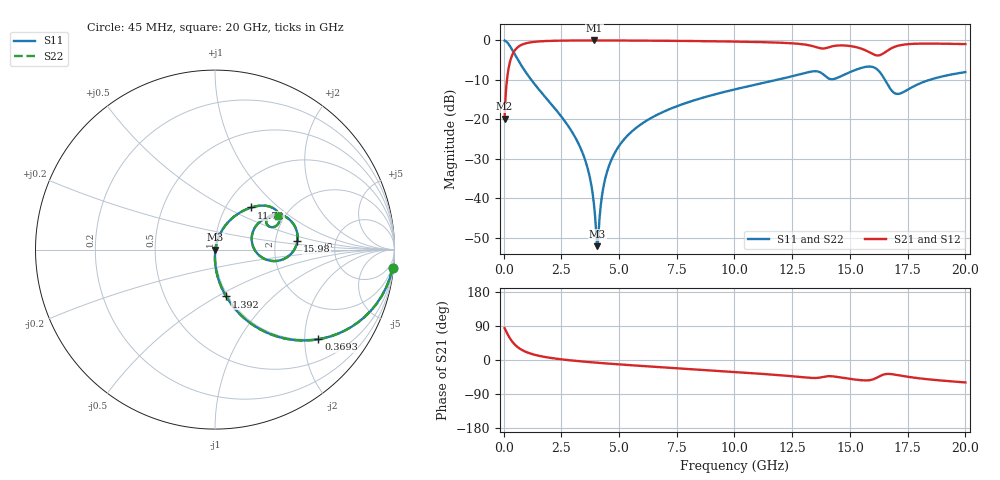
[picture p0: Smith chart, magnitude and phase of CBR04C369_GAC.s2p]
! S-parameter model data by Modelithics Inc.  support@modelithics.com 813-866-6335  Tampa FL USA
! S-Parameter data specifications:
! Substrate: 20-mil Rogers 4350B, substrate thickness, H=0.508mm, Dielectric constant, Er=3.75
! PCB Mounting Pad Footprint: Pad width, PadW=0.52mm , Pad length, PadL=0.52mm , Pad gap, PadG (edge-to-edge)=0.28mm , Reference planes=1.32mm apart
#  GHz  S  MA  R 50
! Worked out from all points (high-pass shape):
!   801 points, 45 MHz to 20 GHz, reference 50 ohm
!   highest |S21| = -0.02 dB at 3.936 GHz (marker M1); lowest = -19.8 dB at 45 MHz (marker M2)
!   |S21| within 3 dB of the highest: 433.5 MHz to 15.84 GHz (15.41 GHz wide, 189 % of centre); 16.52 GHz to end of sweep
!   lowest |S11| = -52.1 dB at 4.061 GHz (marker M3), VSWR 1.00, Z = 50.2 - j0.0389 ohm
!   |S11| at or under -10 dB: 1.202 GHz to 11.83 GHz (10.63 GHz wide, 163 % of centre); 16.52 GHz to 18.45 GHz (1.929 GHz wide, 11 % of centre)
!   |S22| runs from -52.1 to 0.0 dB; largest |S21 - S12| = 0
!   S11 on the Smith chart (normalised r, x): 45 MHz: 1, -19; 369.3 MHz: 0.97, -2.33; 1.392 GHz: 0.98, -0.55; 11.72 GHz: 1.31, +0.68; 15.98 GHz: 2.67, +0.32; 20 GHz: 1.85, +0.81
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0.045  0.9948 -5.9  0.102 84.1  0.102 84.1  0.9948 -5.9
0.219606  0.8937 -27.0  0.4484 62.9  0.4484 62.9  0.8937 -27.0
0.369269  0.7624 -40.9  0.6466 49.0  0.6466 49.0  0.7624 -40.9
0.768369  0.4822 -62.4  0.875 27.5  0.875 27.5  0.4822 -62.4
1.391962  0.2682 -76.6  0.9619 13.1  0.9619 13.1  0.2682 -76.6
3.387462  0.03982 -90.5  0.9968 -3.8  0.9968 -3.8  0.03982 -90.5
3.736675  0.01841 -88.2  0.9973 -5.6  0.9973 -5.6  0.01841 -88.2
3.936225  0.007312 -77.1  0.9974 -6.6  0.9974 -6.6  0.007312 -77.1
4.060944  0.002488 -8.9  0.9974 -7.3  0.9974 -7.3  0.002488 -8.9
4.385212  0.01698 72.4  0.9971 -8.8  0.9971 -8.8  0.01698 72.4
4.784313  0.03621 75.1  0.9965 -10.6  0.9965 -10.6  0.03621 75.1
5.532625  0.06939 73.7  0.9945 -13.9  0.9945 -13.9  0.06939 73.7
6.704981  0.1165 69.7  0.9897 -18.7  0.9897 -18.7  0.1165 69.7
10.0225  0.24 56.9  0.9651 -31.8  0.9651 -31.8  0.24 56.9
11.71867  0.3107 49.1  0.94 -39.0  0.94 -39.0  0.3107 49.1
13.36496  0.4042 33.0  0.8488 -47.3  0.8488 -47.3  0.4042 33.0
14.26294  0.3226 27.3  0.8444 -43.2  0.8444 -43.2  0.3226 27.3
15.23574  0.4224 26.7  0.8248 -51.7  0.8248 -51.7  0.4224 26.7
15.98406  0.4611 5.9  0.6717 -51.4  0.6717 -51.4  0.4611 5.9
16.68248  0.261 -9.1  0.7609 -36.8  0.7609 -36.8  0.261 -9.1
17.13147  0.211 13.9  0.8618 -40.5  0.8618 -40.5  0.211 13.9
20  0.3972 27.8  0.8965 -59.2  0.8965 -59.2  0.3972 27.8
